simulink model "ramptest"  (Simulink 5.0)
settings: Solver=ode45  StartTime=0.0  StopTime=200  RelTol=1e-3

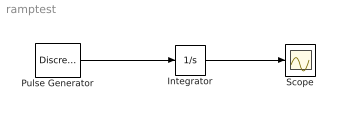
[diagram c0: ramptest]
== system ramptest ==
  Integrator : Integrator
  Pulse Generator : DiscretePulseGenerator  PulseType=Time based  Period=200  PulseWidth=60  PhaseDelay=5
  Scope : Scope
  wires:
  Pulse Generator/1 -> Integrator/1
  Integrator/1 -> Scope/1
